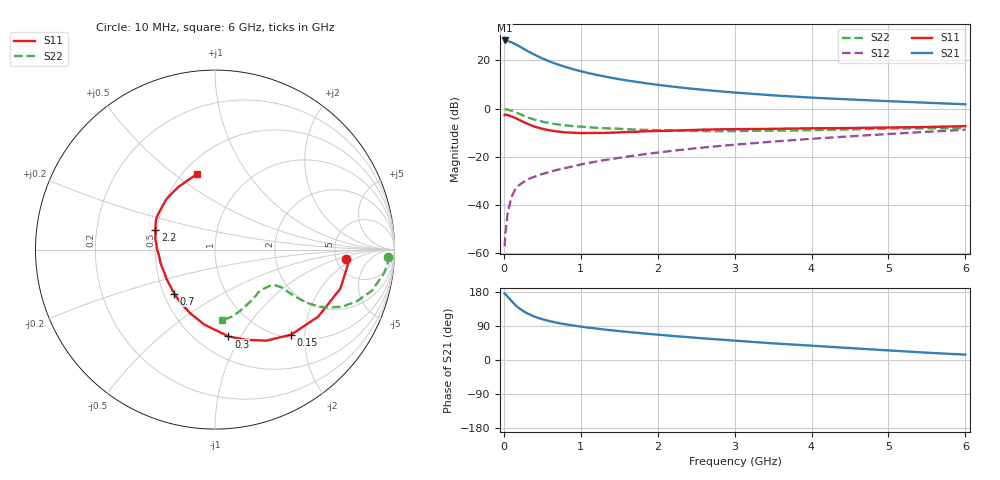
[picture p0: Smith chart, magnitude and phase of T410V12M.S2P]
! Infineon Technologies  Discrete & RF Semiconductors
! BFR182T
! Si NPN RF Bipolar Junction Transistor in SC75
! VCE = 10 V  IC = 12 mA
! Common Emitter S-Parameters:  October  1999
# GHz  S  MA  R  50
!  f  S11  S21  S12  S22
! GHz  MAG  ANG  MAG  ANG  MAG  ANG  MAG  ANG
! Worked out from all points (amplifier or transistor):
!   36 points, 10 MHz to 6 GHz, reference 50 ohm
!   highest |S21| = 28.2 dB at 10 MHz (marker M1)
!   |S21| within 3 dB of that: start of sweep to 232.6 MHz
!   unconditionally stable (mu >= 1): 1.06 GHz to 4.035 GHz
!   at 250 MHz: K = 0.47, MSG = 27.8 dB, |S12| = -30.6 dB
!   at 1.4 GHz: K = 1.06, MAG = 15.4 dB, |S12| = -20.9 dB
!   at 6 GHz: K = 0.87, MSG = 5.3 dB, |S12| = -8.8 dB
!   S11 on the Smith chart (normalised r, x): 10 MHz: 6.18, -1.48; 150 MHz: 1.07, -1.71; 300 MHz: 0.70, -0.89; 700 MHz: 0.57, -0.31; 2.2 GHz: 0.49, +0.12; 6 GHz: 0.59, +0.60
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0.01  0.7347 -4.3  25.85 175.6  0.0014 70.6  0.9621 -2.3
0.02  0.7477 -5.5  25.78 174.3  0.0025 92.2  0.972 -3.1
0.05  0.7315 -17.3  25.21 166.8  0.0069 83.9  0.9519 -7.8
0.1  0.686 -32.9  23.61 155.5  0.0148 73.7  0.9035 -14.7
0.15  0.6365 -48.1  21.69 144.9  0.0214 68.1  0.84 -20.1
0.2  0.5828 -60.5  19.63 136.4  0.0259 67.3  0.7784 -24.1
0.25  0.5308 -71.2  17.62 129.4  0.0295 62.0  0.717 -26.7
0.3  0.4893 -81.2  15.87 123.5  0.0336 62.1  0.668 -28.5
0.4  0.4217 -98.3  13.07 114.1  0.0387 59.6  0.5877 -30.2
0.5  0.3797 -111.6  10.98 107.6  0.0439 60.1  0.5358 -30.3
0.6  0.3523 -123.2  9.41 102.3  0.0488 60.3  0.498 -30.3
0.7  0.3343 -132.9  8.241 97.9  0.0539 61.6  0.4692 -30.0
0.9  0.3153 -149.3  6.555 91.1  0.0634 63.4  0.4315 -29.8
1.1  0.311 -161.9  5.454 85.3  0.0743 64.3  0.4099 -30.1
1.3  0.313 -171.7  4.669 80.6  0.085 65.1  0.392 -30.8
1.6  0.326 176.7  3.828 74.2  0.1005 65.8  0.3732 -32.5
2.2  0.3493 161.9  2.844 63.4  0.1336 65.6  0.3506 -38.1
2.8  0.3709 151.2  2.286 54.0  0.1668 64.3  0.3387 -45.0
3.5  0.3797 140.6  1.879 43.9  0.2063 61.9  0.3486 -54.0
4.5  0.3947 127.7  1.544 31.5  0.2655 57.5  0.3693 -68.1
5.5  0.415 111.4  1.319 19.3  0.3294 52.3  0.39 -79.9
6  0.4319 103.6  1.227 14.1  0.3638 48.9  0.3917 -84.6
